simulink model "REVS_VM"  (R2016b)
settings: Solver=ode3  StartTime=REVS.sim_start_time_secs  StopTime=Inf  FixedStep=REVS.sim_step_time_secs  MaxStep=REVS.sim_step_time_secs  EnableMultiTasking=on
StopFcn:
  | postproc_datalog;
  | postproc_audit;
  | postproc_result;
model workspace (MATLAB code in the model file):
  other statements: REVS_setup_variants
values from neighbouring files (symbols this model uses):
  accessory = class_accessory_data    [class_test_data.m]
  battery = class_battery_data    [class_accessory_data.m]    (also in class_REVS_electric.m = class_REVS_battery)
  brake = struct(	'max_torque_Nm',[], 						'proportion_norm',1.0, 						'inertia_kgm2',0.0)    [class_REVS_drive_axle.m]
  engine = class_engine_data    [class_test_data.m]
  final_drive = struct(	'gear_ratio',[], 								'efficiency_norm',[], 								'inertia_kgm2',[] )    [class_REVS_drive_axle.m]
  gear = class_REVS_gearbox    [class_REVS_AT_transmission.m]
  tire = struct(	'radius_m',[], 						'rolling_resistance_coefficient',0, 						'vehicle_weight_norm',1.0,  						'wheel_slip_torque_Nm',[],  						'inertia_kgm2',0.0)    [class_REVS_drive_axle.m]
  torque_converter = class_REVS_torque_converter    [class_REVS_AT_transmission.m]
  transmission = class_transmission_data    [class_test_data.m]
  vehicle = class_vehicle_data    [class_test_data.m]
undefined symbols (not defined in the file or in its folder): alternator, ambient, controls, convert, DelayTimeSecs, drive_cycle, driver, electric, gear_strategy, InitialCondition, InitialValue, LoadSource, LookupStructure, MultiplyPosInputs, Normalize, NumPhases, REVS, SpeedSource, starter, tableshift, UpperSaturationLimit, Value, VerboseLevel, VerboseSignal
libraries: simulink x153
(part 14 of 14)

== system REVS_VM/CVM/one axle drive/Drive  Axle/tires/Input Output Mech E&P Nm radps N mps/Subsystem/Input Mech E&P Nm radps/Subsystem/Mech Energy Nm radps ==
  trq_Nm : Inport
  spd_radps : Inport  Port=2
  Gain : Gain  Gain=-1
  Integrator : Integrator  ZeroCross=off
  Integrator1 : Integrator  ZeroCross=off
  Integrator2 : Integrator  ZeroCross=off
  Mux : Mux  Inputs=2
  Neg : Fcn  Expr=u(1)*(u(1) <= 0)
  Pos : Fcn  Expr=u(1)*(u(1) >= 0)
  calc_Power_kW : Fcn  Expr=u(1)*u(2)/1000
  "total_kJ " : Outport
  "pos_kJ " : Outport  Port=2
  neg_kJ : Outport  Port=3
  pwr_kW : Outport  Port=4
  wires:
  calc_Power_kW/1 -> Pos/1, Neg/1, pwr_kW/1, Integrator/1
  Gain/1 -> neg_kJ/1
  Integrator1/1 -> "pos_kJ "/1
  Integrator2/1 -> Gain/1
  Neg/1 -> Integrator2/1
  Pos/1 -> Integrator1/1
  spd_radps/1 -> Mux/2
  trq_Nm/1 -> Mux/1
  Mux/1 -> calc_Power_kW/1
  Integrator/1 -> "total_kJ "/1

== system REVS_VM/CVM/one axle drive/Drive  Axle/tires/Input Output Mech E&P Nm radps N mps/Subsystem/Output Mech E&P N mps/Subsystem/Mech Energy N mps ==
  force_N : Inport
  spd_mps : Inport  Port=2
  Gain : Gain  Gain=-1
  Integrator : Integrator  ZeroCross=off
  Integrator1 : Integrator  ZeroCross=off
  Integrator2 : Integrator  ZeroCross=off
  Mux : Mux  Inputs=2
  Neg : Fcn  Expr=u(1)*(u(1) <= 0)
  Pos : Fcn  Expr=u(1)*(u(1) >= 0)
  calc_Power_kW : Fcn  Expr=u(1)*u(2)/1000
  "total_kJ " : Outport
  "pos_kJ " : Outport  Port=2
  neg_kJ : Outport  Port=3
  pwr_kW : Outport  Port=4
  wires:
  calc_Power_kW/1 -> Pos/1, Neg/1, pwr_kW/1, Integrator/1
  Gain/1 -> neg_kJ/1
  Integrator1/1 -> "pos_kJ "/1
  Integrator2/1 -> Gain/1
  Neg/1 -> Integrator2/1
  Pos/1 -> Integrator1/1
  Integrator/1 -> "total_kJ "/1
  Mux/1 -> calc_Power_kW/1
  force_N/1 -> Mux/1
  spd_mps/1 -> Mux/2

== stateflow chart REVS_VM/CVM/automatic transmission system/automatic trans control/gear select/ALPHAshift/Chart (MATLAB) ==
  state gear_command_timer
    entry:
    command_gear_num = launch_gear_num;
    shift_delay_timer = 0;
    in_gear_timer = 0;
    previous_shift_type = -1;
    during:
    % update timers
    shift_delay_timer = shift_delay_timer + dt;
    in_gear_timer = in_gear_timer + dt;
    state downshift_delay
    state upshift_delay
    state in_gear
      exit:
      shift_delay_timer = 0;
    (default) -> in_gear
    in_gear -> upshift_delay : [desired_gear_num > command_gear_num]
    in_gear -> downshift_delay : [desired_gear_num < command_gear_num]
    upshift_delay -> in_gear : [desired_gear_num <= command_gear_num]
    downshift_delay -> in_gear : [desired_gear_num >= command_gear_num]
    upshift_delay -> in_gear : [(shift_delay_timer >= upshift_delay_secs && ... (in_gear_timer > downshift_min_duration_secs && previous_shift_type == -1 || ... in_gear_timer > upshift_min_duration_secs && previous_shift_type == +1) ) || ... (shift_delay_timer >= upshift_delay_secs/10 && desired_shift_reason == 4)]   {command_gear_num = desired_gear_num; in_gear_timer = 0; previous_shift_type = +1; shift_reason = desired_shift_reason}
    downshift_delay -> in_gear : [shift_delay_timer >= downshift_delay_secs && ... (in_gear_timer > downshift_min_duration_secs && previous_shift_type == -1 || ... in_gear_timer > upshift_min_duration_secs && previous_shift_type == +1) || ... legacy_downshift_mode && (desired_shift_reason ~= 3) ]    {command_gear_num = desired_gear_num; in_gear_timer = 0; previous_shift_type = -1; shift_reason = desired_shift_reason}
  (default) -> gear_command_timer
  data: dt input; command_gear_num output; previous_shift_type output; downshift_min_duration_secs input; upshift_min_duration_secs input; launch_gear_num input; upshift_delay_secs input; desired_gear_num input; downshift_delay_secs input; legacy_downshift_mode input; shift_reason output; shift_delay_timer output; desired_shift_reason input; in_gear_timer output

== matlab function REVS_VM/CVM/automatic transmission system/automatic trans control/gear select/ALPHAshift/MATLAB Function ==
 function [  desired_gear_num, ...
            desired_shift_reason, ...
            kickdown_timer, ...
            kickdown_ratio, ...
            gear_available, ...
            gear_disability_code, ...
            better_cost_gear, ...
            min_cost_gear, ... 
   kickdown_gear_available, ...
            kickdown_disability_code ...
          ] = ...
fcn(gear_strategy, ...
    desired_shift_reason_prev, ...
    kickdown_timer_prev, ...
    kickdown_ratio_prev, ...
    command_gear_num, ...
    current_gear_num, ...
    dt, ...
    vehicle_spd_mps, ...
    driver_des_pwr_W, ...
    engine_max_pwr_W, ...
    gear_trq_Nm, ...
    gear_spd_radps, ...
    gear_cost, ...
    gear_avail_trq_Nm) ...

% entry:
desired_shift_reason    = desired_shift_reason_prev;
kickdown_timer          = kickdown_timer_prev;
current_gear_index      = current_gear_num+1;
desired_gear_num        = current_gear_num; % init desired gear to current gear

num_gear_indices = length( gear_avail_trq_Nm );
gear_indices = reshape((1:num_gear_indices), size(gear_avail_trq_Nm));
gear_nums = gear_indices-1;

gear_avail_trq_Nm = gear_avail_trq_Nm .* (gear_nums > 0); % no torque available in neutral

% define which gears meet speed and torque boundary conditions:
gear_disability_code =  (gear_spd_radps < gear_strategy.min_speed_radps) * 1 + ...
                        (gear_spd_radps > gear_strategy.max_speed_radps) * 2 + ...
                        (gear_avail_trq_Nm < gear_trq_Nm) * 4 + ...
                        ((gear_nums > current_gear_num) & (gear_spd_radps < gear_strategy.upshift_min_speed_radps)) * 8 + ...
                        ((gear_nums > current_gear_num) & (gear_avail_trq_Nm < (gear_trq_Nm * gear_strategy.upshift_min_torque_reserve_ratio(current_gear_index)))) * 16 + ...
                        ((gear_nums < current_gear_num) & (gear_spd_radps > gear_strategy.downshift_max_speed_radps)) * 32 + ...;
                        (gear_strategy.restrict_skip_shifts & (abs(current_gear_num - gear_nums) > 1)) * 64 + ...
                        (gear_strategy.restrict_shift_parity & (mod(gear_nums,2) == mod(current_gear_num,2)) & (gear_nums ~= current_gear_num)) * 128 + ...
                        (gear_avail_trq_Nm == 0) * 256;

gear_available = (gear_disability_code == 0);

if isempty(gear_cost(gear_available & (gear_nums > 0)))
    min_fuel_gear_index = 2;
    min_cost_gear = 1;
else
    [~, min_index] = min(gear_cost(gear_available & (gear_nums > 0)));
    gear_indices_available = gear_indices(gear_available  & (gear_nums > 0));
    min_fuel_gear_index = gear_indices_available(min_index);
    min_cost_gear = gear_nums(min_fuel_gear_index);
end

% create binary vector of all gear indices that have better fuel
% cost and meet boundary conditions...
better_cost_gear = gear_available & (gear_cost < (gear_cost(current_gear_index) / gear_strategy.required_cost_benefit_ratio(current_gear_index)));

% calculate non-fuel-based shift points:
kickdown_ratio = max(0,driver_des_pwr_W/max(1,engine_max_pwr_W));
%future_kickdown_ratio = kickdown_ratio + (kickdown_ratio - kickdown_ratio_prev) * 1/dt;

if better_cost_gear(min_fuel_gear_index) && ...
        (min_fuel_gear_index ~= current_gear_index) && ...
        ( kickdown_ratio < gear_strategy.kickdown_trigger_ratio(current_gear_index) )
    if (min_fuel_gear_index > current_gear_index)
        desired_gear_num = min_cost_gear;
        desired_shift_reason = 1 + gear_disability_code(current_gear_index)/10;
    elseif (min_fuel_gear_index < current_gear_index) && (gear_strategy.disable_cost_saving_downshifts == false)
        desired_gear_num = min_cost_gear;
        desired_shift_reason = 2 + gear_disability_code(current_gear_index)/10;
    end
end

% 	(gear_strategy.restrict_skip_shifts & (abs(current_gear_num - gear_nums) > 1)) * 64 + ...	% Shared with codes above
kickdown_disability_code = ...
    (gear_spd_radps >= gear_strategy.downshift_max_speed_radps) * 32 + ...	% Shared with codes above
    (gear_strategy.restrict_shift_parity & (mod(gear_nums,2) == mod(current_gear_num,2))) * 128 + ...;	% Shared with codes above
	(gear_nums < (current_gear_num - gear_strategy.kickdown_max_increment)) * 256 + ...
    (gear_nums < gear_strategy.kickdown_min_gear) * 512 +...
	(gear_nums >= current_gear_num) * 1024;
kickdown_gear_available = (kickdown_disability_code == 0);

if  ( kickdown_ratio >= gear_strategy.kickdown_trigger_ratio(current_gear_index) ) && any(kickdown_gear_available)
    kickdown_timer = kickdown_timer + dt;
else
    kickdown_timer = 0;
end

if any(kickdown_gear_available ) && kickdown_timer >= gear_strategy.kickdown_delay_secs(current_gear_index)
    
    kickdown_power_available = ((gear_spd_radps .* gear_avail_trq_Nm - driver_des_pwr_W) > 0) & kickdown_gear_available ;
	
	if any(kickdown_power_available )
		desired_gear_num = max( gear_nums( kickdown_power_available ) );
	else
		desired_gear_num = min( gear_nums( kickdown_gear_available ) );
	end
	
    desired_shift_reason = 3;
end

if (gear_spd_radps(current_gear_index) > gear_strategy.max_speed_radps(current_gear_index)) 
	max_speed_upshift_gear_index = min(num_gear_indices, current_gear_index + gear_strategy.max_speed_shift_increment(current_gear_index));
	
	if  (gear_disability_code(max_speed_upshift_gear_index) < 256)
		desired_gear_num = command_gear_num + gear_strategy.max_speed_shift_increment(current_gear_index);
		desired_shift_reason = 4;
	end
end

if (gear_spd_radps(current_gear_index) < gear_strategy.min_speed_radps(current_gear_index)) && ( command_gear_num > gear_strategy.launch_gear_num)
    desired_gear_num = command_gear_num - gear_strategy.min_speed_shift_increment(current_gear_index);
    desired_shift_reason = 5;
end

if vehicle_spd_mps <= 1
    desired_gear_num = gear_strategy.launch_gear_num;
    desired_shift_reason = 6;
end

desired_gear_num = min(num_gear_indices-1 , max(1, desired_gear_num));

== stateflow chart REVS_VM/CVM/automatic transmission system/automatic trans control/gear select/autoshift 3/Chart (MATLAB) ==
  state gear_command_timer
    entry:
    command_gear_num = launch_gear_num;
    shift_delay_timer = 0;
    in_gear_timer = 0;
    previous_shift_type = -1;
    during:
    % update timers
    shift_delay_timer = shift_delay_timer + dt;
    in_gear_timer = in_gear_timer + dt;
    state downshift_delay
    state upshift_delay
    state in_gear
      exit:
      shift_delay_timer = 0;
    (default) -> in_gear
    in_gear -> upshift_delay : [desired_gear_num > command_gear_num]
    in_gear -> downshift_delay : [desired_gear_num < command_gear_num]
    upshift_delay -> in_gear : [desired_gear_num <= command_gear_num]
    downshift_delay -> in_gear : [desired_gear_num >= command_gear_num]
    upshift_delay -> in_gear : [(shift_delay_timer >= upshift_delay_secs && ... (in_gear_timer > downshift_min_duration_secs && previous_shift_type == -1 || ... in_gear_timer > upshift_min_duration_secs && previous_shift_type == +1) ) || ... (shift_delay_timer >= upshift_delay_secs/10 && desired_shift_reason == 4)]   {command_gear_num = desired_gear_num; in_gear_timer = 0; previous_shift_type = +1; shift_reason = desired_shift_reason}
    downshift_delay -> in_gear : [shift_delay_timer >= downshift_delay_secs && ... (in_gear_timer > downshift_min_duration_secs && previous_shift_type == -1 || ... in_gear_timer > upshift_min_duration_secs && previous_shift_type == +1) || ... legacy_downshift_mode && (desired_shift_reason ~= 3) ]    {command_gear_num = desired_gear_num; in_gear_timer = 0; previous_shift_type = -1; shift_reason = desired_shift_reason}
  (default) -> gear_command_timer
  data: dt input; command_gear_num output; previous_shift_type output; downshift_min_duration_secs input; upshift_min_duration_secs input; launch_gear_num input; upshift_delay_secs input; desired_gear_num input; downshift_delay_secs input; legacy_downshift_mode input; shift_reason output; shift_delay_timer output; desired_shift_reason input; in_gear_timer output

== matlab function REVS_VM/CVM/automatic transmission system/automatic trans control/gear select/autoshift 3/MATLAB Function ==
 function [  desired_gear_num, ...
            desired_shift_reason, ...
            kickdown_timer, ...
            kickdown_ratio, ...
            gear_available, ...
            gear_disability_code, ...
            better_cost_gear, ...
            min_cost_gear ... 
          ] = ...
fcn(gear_strategy,  ...
    desired_shift_reason_prev, ...
    kickdown_timer_prev, ...
    kickdown_ratio_prev, ...
    command_gear_num, ...
    current_gear_num, ...
    dt, ...
    vehicle_spd_mps, ...
    driver_des_pwr_W, ...
    engine_max_pwr_W, ...
    gear_trq_Nm, ...
    gear_spd_radps, ...
    gear_cost, ...
    gear_avail_trq_Nm) ...

% entry:
desired_shift_reason    = desired_shift_reason_prev;
kickdown_timer          = kickdown_timer_prev;
current_gear_index      = current_gear_num+1;
desired_gear_num        = current_gear_num; % init desired gear to current gear

num_gear_indices = length( gear_avail_trq_Nm );
gear_indices = (1:num_gear_indices);
gear_nums = gear_indices-1;

gear_avail_trq_Nm = gear_avail_trq_Nm .* (gear_nums > 0); % no torque available in neutral

% define which gears meet speed and torque boundary conditions:
gear_disability_code =  (gear_spd_radps < gear_strategy.min_speed_radps) * 1 + ...
                        (gear_spd_radps > gear_strategy.max_speed_radps) * 2 + ...
                        (gear_avail_trq_Nm < gear_trq_Nm) * 4 + ...
                        ((gear_nums > current_gear_num) & (gear_spd_radps < gear_strategy.upshift_min_speed_radps)) * 8 + ...
                        ((gear_nums > current_gear_num) & (gear_avail_trq_Nm < (gear_trq_Nm * gear_strategy.upshift_min_torque_reserve_ratio(current_gear_index)))) * 16 + ...
                        ((gear_nums < current_gear_num) & (gear_spd_radps > gear_strategy.downshift_max_speed_radps)) * 32 + ...;
                        (gear_strategy.restrict_skip_shifts & (abs(current_gear_num - gear_nums) > 1)) * 64 + ...
                        (gear_strategy.restrict_shift_parity & (mod(gear_nums,2) == mod(current_gear_num,2)) & (gear_nums ~= current_gear_num)) * 128 + ...
                        (gear_avail_trq_Nm == 0) * 256;

gear_available = (gear_disability_code == 0);

if isempty(gear_cost(gear_available & (gear_nums > 0)))
    min_fuel_gear_index = 2;
    min_cost_gear = 1;
else
    [~, min_index] = min(gear_cost(gear_available & (gear_nums > 0)));
    gear_indices_available = gear_indices(gear_available  & (gear_nums > 0));
    min_fuel_gear_index = gear_indices_available(min_index);
    min_cost_gear = gear_nums(min_fuel_gear_index);
end

% create binary vector of all gear indices that have better fuel
% cost and meet boundary conditions...
better_cost_gear = gear_available & (gear_cost < (gear_cost(current_gear_index) / gear_strategy.required_cost_benefit_ratio(current_gear_index)));

if better_cost_gear(min_fuel_gear_index) && (min_fuel_gear_index ~= current_gear_index)
    if (min_fuel_gear_index > current_gear_index)
        desired_gear_num = min_cost_gear;
        desired_shift_reason = 1 + gear_disability_code(current_gear_index)/10;
    elseif (min_fuel_gear_index < current_gear_index) && (gear_strategy.disable_cost_saving_downshifts == false)
        desired_gear_num = min_cost_gear;
        desired_shift_reason = 2 + gear_disability_code(current_gear_index)/10;
    end
end

% calculate non-fuel-based shift points:
kickdown_ratio = driver_des_pwr_W/max(1,engine_max_pwr_W);
future_kickdown_ratio = kickdown_ratio + (kickdown_ratio - kickdown_ratio_prev) * 1/dt;
%if gear_engine_torque_Nm(current_gear_index) / gear_available_torque_Nm(current_gear_index) > 0.999  && (gear_engine_speed_radps(current_gear_index - 1) < max_engine_spd_radps * 0.85)
%if (driver_des_pwr_W > (engine_max_pwr_W * min_available_torque_reserve_ratio))  && (gear_engine_speed_radps(current_gear_index - 1) < max_engine_spd_radps * 0.85)

%%        (kickdown_ratio >= kickdown_ratio_prev * 0.99/0.99)  && ...

if ( current_gear_index - 1 > 1) && ...
    ( kickdown_ratio >= gear_strategy.kickdown_trigger_ratio(current_gear_index) ) && ...
	( future_kickdown_ratio >= gear_strategy.kickdown_trigger_ratio(current_gear_index) ) && ...
	( gear_spd_radps(current_gear_index - 1) < gear_strategy.downshift_max_speed_radps(current_gear_index-1))
    kickdown_timer = kickdown_timer + dt;
else
%    if (kickdown_ratio < 1.0)
        kickdown_timer = 0;
%    else
%        kickdown_timer = max(0, kickdown_timer - dt);
%    end
end

if (kickdown_timer >= gear_strategy.kickdown_delay_secs(current_gear_index)) && (command_gear_num > 1)
    desired_gear_num = command_gear_num - 1;
    desired_shift_reason = 3;
end

%if (gear_spd_radps(current_gear_index) > gear_strategy.max_speed_radps(current_gear_index)) && ...
%        (gear_available(min(num_gear_indices, current_gear_index + gear_strategy.max_speed_shift_increment(current_gear_index))))
if (gear_spd_radps(current_gear_index) > gear_strategy.max_speed_radps(current_gear_index)) && ...
        (gear_disability_code(min(num_gear_indices, current_gear_index + gear_strategy.max_speed_shift_increment(current_gear_index))) < 256)
    desired_gear_num = command_gear_num + gear_strategy.max_speed_shift_increment(current_gear_index);
    desired_shift_reason = 4;
end

if (gear_spd_radps(current_gear_index) < gear_strategy.min_speed_radps(current_gear_index)) && ... 
        ( command_gear_num > gear_strategy.launch_gear_num) && ...
        ( gear_spd_radps(current_gear_index - gear_strategy.min_speed_shift_increment(current_gear_index)) < gear_strategy.downshift_max_speed_radps(current_gear_index - gear_strategy.min_speed_shift_increment(current_gear_index)))
    desired_gear_num = command_gear_num - gear_strategy.min_speed_shift_increment(current_gear_index);
    desired_shift_reason = 5;
end

if vehicle_spd_mps <= 1
    desired_gear_num = gear_strategy.launch_gear_num;
    desired_shift_reason = 6;
end

desired_gear_num = min(num_gear_indices-1 , max(1, desired_gear_num));

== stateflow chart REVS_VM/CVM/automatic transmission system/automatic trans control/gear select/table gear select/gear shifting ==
  state Upshift_delay
    entry:
    timer = 0;
    during:
    timer += step_time;
  state In_gear
    entry:
    during:
  state Downshift_delay
    entry:
    timer = 0;
    during:
    timer += step_time;
  (default) -> In_gear : {driver_gear = 1;}
  In_gear -> Downshift_delay : [(shift_spd <= downshift_spd) ]
  In_gear -> Upshift_delay : [(shift_spd >= upshift_spd)]
  Downshift_delay -> In_gear : [(shift_spd > downshift_spd)]
  Upshift_delay -> In_gear : [(shift_spd < upshift_spd)]
  Downshift_delay -> In_gear : [(shift_spd <= downshift_spd) && (timer >=  0.01) &&...  (timer >=  downshift_delay_secs) && (driver_gear > 1)]  {driver_gear = max(1, driver_gear-1);}
  Upshift_delay -> In_gear : [(shift_spd > upshift_spd) &&  (timer >=  upshift_delay_secs)]  {driver_gear = max(1, driver_gear+1);}
  data: shift_spd input double; driver_gear output double; step_time input double; upshift_delay_secs input double; upshift_spd input double; downshift_spd input double; timer local double; downshift_delay_secs input double

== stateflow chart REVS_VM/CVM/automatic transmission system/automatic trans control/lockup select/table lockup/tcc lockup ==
  state TCC_OFF
    entry:
    tcc_lockup = false;
    timer = 0;
    during:
    timer += step_time;
  state TCC_ON
    entry:
    tcc_lockup=true;
  (default) -> TCC_OFF
  TCC_OFF -> TCC_OFF : [lock_spd < lockup_spd || ... ~lockup_allowed]
  TCC_OFF -> TCC_ON : [lockup_allowed && ... (lock_spd >= lockup_spd) && ...  (timer >= lockup_delay_secs)]
  TCC_ON -> TCC_OFF : [lock_spd <= release_spd]
  data: lock_spd input; step_time input; lockup_spd input double; release_spd input double; tcc_lockup output double; timer local double; lockup_allowed input; lockup_delay_secs input
